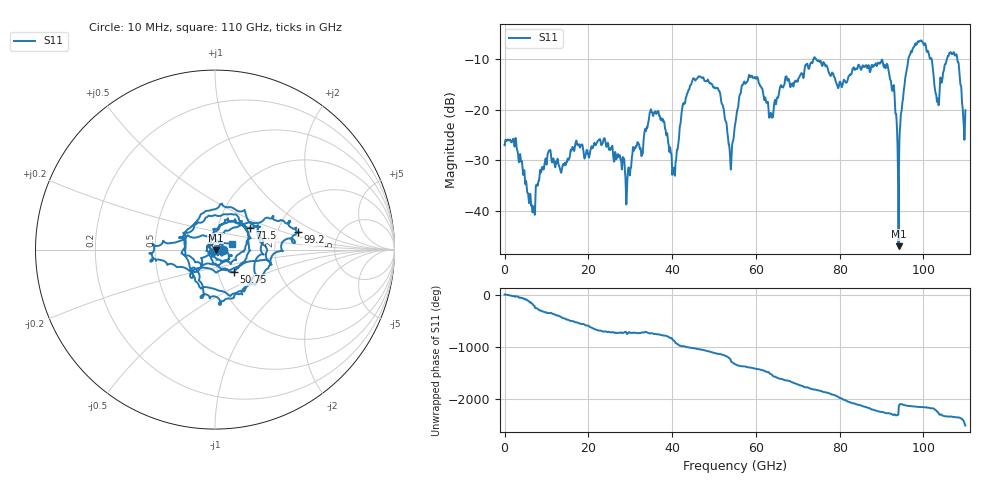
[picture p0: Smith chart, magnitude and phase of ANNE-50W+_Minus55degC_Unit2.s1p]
!Mini-Circuits Laboratory
!S-Parameters
!S1P File: Measurement
!Model: ANNE-50W+
!No.: Unit# 2 (U2_-55°C)
!Run / Lot / Date Code: QN2409253 /  / 2409
!Fixture: N/A
!Network Analyzer: PNA-X N5242B;  Serial number: 74314
!Pin Outs: PORT<1> = pin<1>
!TEST CONDITIONS: Z:50 OHM SYSTEM, INPUT POWER = 0dBm, TEMP:25°C
!F-F adapter to 1FT F-M cable on Port 2 head. 1mm 1 PORT SmartCal
!Date: 9/5/2024 at 12:58:10 PM
# Hz  S  dB  R  50
!Frequency  S11 dB  S11 Deg
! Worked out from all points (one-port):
!   2208 points, 10 MHz to 110 GHz, reference 50 ohm
!   lowest |S11| = -46.9 dB at 94.05 GHz (marker M1), VSWR 1.01, Z = 50.4 - j0.278 ohm
!   |S11| at or under -10 dB: start of sweep to 73.79 GHz; 74.17 GHz to 96.4 GHz (22.23 GHz wide, 26.1 % of centre); 101.9 GHz to 105.6 GHz (3.709 GHz wide, 3.57 % of centre)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
!   S11 on the Smith chart (normalised r, x): 10 MHz: 1.09, -0.00; 50.75 GHz: 1.19, -0.30; 71.5 GHz: 1.43, +0.37; 99.2 GHz: 2.61, +0.66; 110 GHz: 1.20, +0.08
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1e7  -27.03 -0.3
6.8e9  -39.51 161.4
1.055e10  -28.15 5.7
1.38e10  -31.25 -85.7
2.755e10  -29.04 -7.3
2.945e10  -32.03 -18.2
3.52e10  -20.62 -20.3
4.035e10  -31.75 -156.4
4.13e10  -27.82 135.0
4.48e10  -14.41 57.1
5.075e10  -15.83 -49.9
5.38e10  -28.83 -145.0
5.505e10  -22.81 109.2
5.86e10  -13.60 45.9
6.36e10  -20.67 -81.2
6.88e10  -14.95 121.9
7.15e10  -12.79 31.9
7.66e10  -11.51 -66.9
8.255e10  -13.16 100.7
8.65e10  -11.70 5.5
9.12e10  -11.10 -106.9
9.405e10  -46.86 -37.4
9.63e10  -10.58 31.0
9.92e10  -6.48 11.9
1.0325e11  -18.51 -75.8
1.061e11  -9.08 -171.7
1.0805e11  -9.99 176.2
1.1e11  -20.13 19.8
